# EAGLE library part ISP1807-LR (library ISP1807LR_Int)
ISP Smart Bluetooth Module
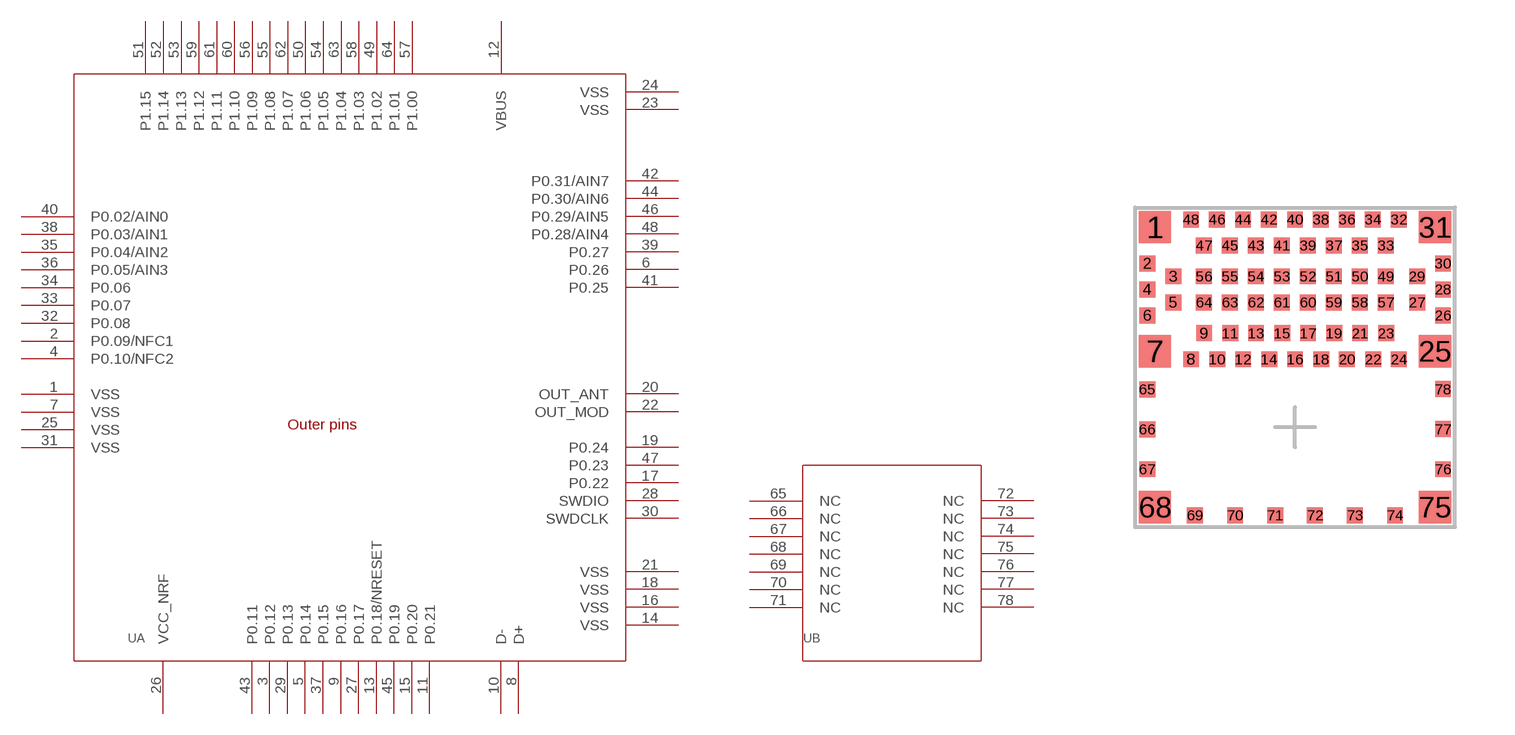
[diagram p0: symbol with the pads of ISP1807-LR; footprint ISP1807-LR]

Designator prefix U; gates A=ISP1807-LR_A B=ISP1807-LR_B

## ISP1807-LRISP1807-LR_ISP1807-LR (BOI: QFN 8 x 8; BOI-METRIC: QFN 8 x 8; DESIG: BLE Module; FAB: Insight SiP; ISP_PART: ISP1807; REF: ISP1807-LR)  [ISP1807-LR]
1  A:VSS  pwr
2  A:P0.09/NFC1
3  A:P0.12
4  A:P0.10/NFC2
5  A:P0.14
6  A:P0.26
7  A:VSS  pwr
8  A:D+  pwr
9  A:P0.16
10  A:D-  pwr
11  A:P0.21
12  A:VBUS  pwr
13  A:P0.18/NRESET
14  A:VSS  pwr
15  A:P0.20
16  A:VSS  pwr
17  A:P0.22
18  A:VSS  pwr
19  A:P0.24
20  A:OUT_ANT
21  A:VSS  pwr
22  A:OUT_MOD
23  A:VSS  pwr
24  A:VSS  pwr
25  A:VSS  pwr
26  A:VCC_NRF  pwr
27  A:P0.17
28  A:SWDIO
29  A:P0.13
30  A:SWDCLK  in
31  A:VSS  pwr
32  A:P0.08
33  A:P0.07
34  A:P0.06
35  A:P0.04/AIN2
36  A:P0.05/AIN3
37  A:P0.15
38  A:P0.03/AIN1
39  A:P0.27
40  A:P0.02/AIN0
41  A:P0.25
42  A:P0.31/AIN7
43  A:P0.11
44  A:P0.30/AIN6
45  A:P0.19
46  A:P0.29/AIN5
47  A:P0.23
48  A:P0.28/AIN4
49  A:P1.02
50  A:P1.06
51  A:P1.15
52  A:P1.14
53  A:P1.13
54  A:P1.05
55  A:P1.08
56  A:P1.09
57  A:P1.00
58  A:P1.03
59  A:P1.12
60  A:P1.10
61  A:P1.11
62  A:P1.07
63  A:P1.04
64  A:P1.01
65  B:NC  pas
66  B:NC  pas
67  B:NC  pas
68  B:NC  pas
69  B:NC  pas
70  B:NC  pas
71  B:NC  pas
72  B:NC  pas
73  B:NC  pas
74  B:NC  pas
75  B:NC  pas
76  B:NC  pas
77  B:NC  pas
78  B:NC  pas

## Footprint ISP1807-LR (pad centres in mm)
smd 0.8 x 0.8: 1 0.5,-0.5; 7 0.5,-3.6; 25 7.5,-3.6; 31 7.5,-0.5; 68 0.5,-7.5; 75 7.5,-7.5
smd 0.4 x 0.4: 2 0.3,-1.4; 3 0.95,-1.725; 4 0.3,-2.05; 5 0.95,-2.375; 6 0.3,-2.7; 8 1.4,-3.8; 9 1.725,-3.15; 10 2.05,-3.8; 11 2.375,-3.15; 12 2.7,-3.8; 13 3.025,-3.15; 14 3.35,-3.8; 15 3.675,-3.15; 16 4,-3.8; 17 4.325,-3.15; 18 4.65,-3.8; 19 4.975,-3.15; 20 5.3,-3.8; 21 5.625,-3.15; 22 5.95,-3.8; 23 6.275,-3.15; 24 6.6,-3.8; 26 7.7,-2.7; 27 7.05,-2.375; 28 7.7,-2.05; 29 7.05,-1.725; 30 7.7,-1.4; 32 6.6,-0.3; 33 6.275,-0.95; 34 5.95,-0.3; 35 5.625,-0.95; 36 5.3,-0.3; 37 4.975,-0.95; 38 4.65,-0.3; 39 4.325,-0.95; 40 4,-0.3; 41 3.675,-0.95; 42 3.35,-0.3; 43 3.025,-0.95; 44 2.7,-0.3; 45 2.375,-0.95; 46 2.05,-0.3; 47 1.725,-0.95; 48 1.4,-0.3; 49 6.275,-1.725; 50 5.625,-1.725; 51 4.975,-1.725; 52 4.325,-1.725; 53 3.675,-1.725; 54 3.025,-1.725; 55 2.375,-1.725; 56 1.725,-1.725; 57 6.275,-2.375; 58 5.625,-2.375; 59 4.975,-2.375; 60 4.325,-2.375; 61 3.675,-2.375; 62 3.025,-2.375; 63 2.375,-2.375; 64 1.725,-2.375; 65 0.3,-4.55; 66 0.3,-5.55; 67 0.3,-6.55; 69 1.5,-7.701; 70 2.5,-7.701; 71 3.5,-7.701; 72 4.5,-7.701; 73 5.5,-7.701; 74 6.5,-7.701; 76 7.7,-6.55; 77 7.7,-5.55; 78 7.7,-4.55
